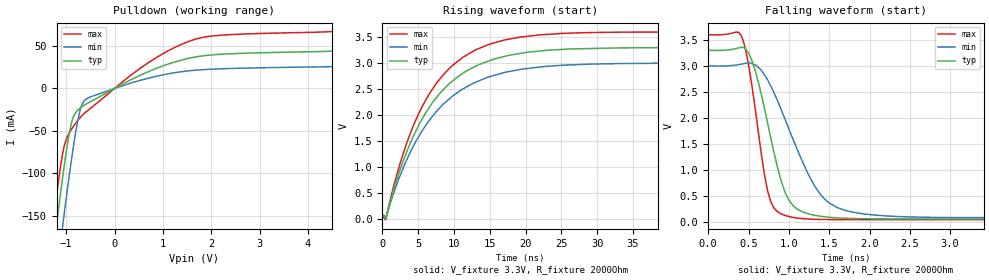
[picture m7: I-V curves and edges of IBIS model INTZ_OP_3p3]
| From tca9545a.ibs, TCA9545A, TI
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|   Model
[Model]   INTZ_OP_3p3
Model_type   Open_drain
Polarity   Non-Inverting
Vmeas = 1.65
Vref = 3.3
Cref = 1pF
Rref = 2000
|   typ   min   max
C_comp   1.601pF   1.487pF   1.862pF
[Voltage Range]   3.3   3   3.6
[Temperature Range]   27   125   -40
[Pullup Reference]   3.3   3   3.6
[Pulldown Reference]   -0   -0   -0
[Power Clamp Reference]   3.3   3   3.6
[GND Clamp Reference]   -0   -0   -0
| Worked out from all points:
|   slope of the pulldown table from 0 to 0.495 V, typ, clamps not added: 33.8 ohm
|   falling waveform, V_fixture 3.3V, R_fixture 2000Ohm: 20-80 % time 296ps typ, 496ps min, 202ps max; typ from 3.3 V to 0.051 V
|   rising waveform, V_fixture 3.3V, R_fixture 2000Ohm: 20-80 % time 7.84ns typ, 8.3ns min, 7.48ns max; typ from 0.051 V to 3.3 V
[Pulldown]
|   Voltage   I(typ)   I(min)   I(max)
-3.3V     -1.182A    -1.239A    -1.147A
-1.29V    -202.2mA   -261.9mA   -166mA
-1.231V   -174.8mA   -234.2mA   -139.4mA
-1.063V   -100.4mA   -157.5mA   -73.82mA
-933.9mV  -52.03mA   -101.8mA   -52.28mA
-864.6mV  -35.35mA   -73.8mA    -45.91mA
-716.1mV  -23.35mA   -26.46mA   -34.59mA
-617.1mV  -19.45mA   -13.84mA   -28.98mA
561mV     16.38mA    10.05mA    25.06mA
1.403V    33.82mA    19.97mA    52.54mA
2.224V    40.48mA    23.29mA    63.01mA
6.59V     47.2mA     28.11mA    71.43mA
[Ramp]
R_load = 2000
|   typ   min   max
dV/dt_r   1.94938/7.83908e-09   1.75549/8.30299e-09   2.13797/7.48178e-09
dV/dt_f   1.9494/2.95962e-10   1.75551/4.95645e-10   2.13799/2.02292e-10
[Falling Waveform]
V_fixture = 3.3V
V_fixture_min = 3V
V_fixture_max = 3.6V
R_fixture = 2000Ohm
C_fixture = 0F
|   Time   V(typ)   V(min)   V(max)
0s        3.3V       3V         3.6V
429.2ps   3.358V     3.04V      3.507V
575.6ps   2.946V     3.024V     2.255V
699.7ps   2.165V     2.821V     885.7mV
811.8ps   1.357V     2.498V     270.2mV
995.1ps   426.9mV    1.804V     100.4mV
1.4ns     100.4mV    504.2mV    40.87mV
1.819ns   58.92mV    173.6mV    37.16mV
3.114ns   51.18mV    76.81mV    36.87mV
100ns     51mV       74.15mV    36.68mV
[Rising Waveform]
V_fixture = 3.3V
V_fixture_min = 3V
V_fixture_max = 3.6V
R_fixture = 2000Ohm
C_fixture = 0F
|   Time   V(typ)   V(min)   V(max)
0s        51mV       74.15mV    36.68mV
478.8ps   18.57mV    51.09mV    -2.274mV
2.163ns   818.1mV    724.8mV    924.5mV
4.381ns   1.61V      1.417V     1.816V
7.535ns   2.335V     2.069V     2.612V
11.27ns   2.808V     2.506V     3.116V
17.05ns   3.131V     2.822V     3.447V
22.98ns   3.248V     2.94V      3.554V
33.67ns   3.296V     2.994V     3.597V
100ns     3.3V       3V         3.6V
